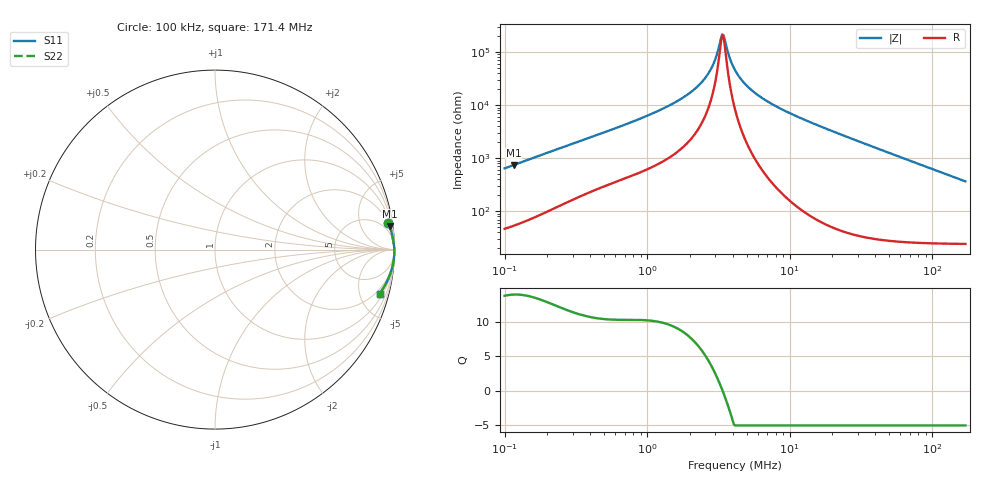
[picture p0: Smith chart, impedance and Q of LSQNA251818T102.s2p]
! LSQNA251818T102  S-PARAMETER MODEL  ( General Type )
! Model Generated by TAIYO YUDEN Corporation (http://www.ty-top.com)
! Version 2.0
! TAIYO YUDEN Control No. 100810NF25SB-FKC
! Copyright(c) 2007 TAIYO YUDEN CO.,LTD. All Rights Reserved.
! Product Description (link to TY-COMPAS)
! https://ds.yuden.co.jp/TYCOMPAS/or/detail?pn=LSQNA251818T102K&u=M
! Products Name : Inductors
! Characteristics :
!  Inductance : 1000 uH , SRF(min) : 2.4 MHz , DC Resistance(max) : 31.2 Ohm
!  Rated Current : Saturation :25 mA , Temp Rise : 75 mA (40 degC)
!  Case Size : 2.5 x 1.8 / 0.098 x 0.071 [mm/inch] , Thickness : 1.8 / 0.071 [mm/inch]
!  (Conditions: Temperature = 25 degC , DC Bias Current/Voltage = 0A / 0V)
! External Node Assignments :
!  1  o---GGG---o  2
! GND o---------o GND
! Frequency Range : 0.1MHz  -  171.398534MHz  [ 402 STEP ]
# MHz S RI R 50
! Freq[MHz].  S11 Real  S11 Imag  S21 Real  S21 Imag  S12 Real  S12 Imag  S22 Real  S22 Imag
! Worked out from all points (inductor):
!   401 points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, 100 kHz to 171.4 MHz, reference 50 ohm
!   read as one part in series: L = 1.02 mH near 103.8 kHz
!   highest Q = 13.9 at 116.1 kHz (marker M1), where L = 1.02 mH
!   self-resonance near 3.373 MHz
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0.1  0.9662 0.1479  0.0338 -0.1479  0.0338 -0.1479  0.9662 0.1479
0.116059  0.9734 0.1289  0.0266 -0.1289  0.0266 -0.1289  0.9734 0.1289
0.348094  0.9937 0.0455  0.00627 -0.0455  0.00627 -0.0455  0.9937 0.0455
1.211692  0.9986 0.0125  0.00142 -0.0125  0.00142 -0.0125  0.9986 0.0125
1.859293  0.9991 0.00668  0.000853 -0.00668  0.000853 -0.00668  0.9991 0.00668
2.157883  0.9993 0.00492  0.000721 -0.00492  0.000721 -0.00492  0.9993 0.00492
2.458233  0.9994 0.00346  0.000626 -0.00346  0.000626 -0.00346  0.9994 0.00346
2.698039  0.9994 0.00244  0.000569 -0.00244  0.000569 -0.00244  0.9994 0.00244
2.90662  0.9995 0.00164  0.000529 -0.00164  0.000529 -0.00164  0.9995 0.00164
3.073571  0.9995 0.00104  0.000503 -0.00104  0.000503 -0.00104  0.9995 0.00104
3.250112  0.9995 0.000449  0.000479 -0.000449  0.000479 -0.000449  0.9995 0.000449
3.373404  0.9995 5.2e-05  0.000464 -5.2e-05  0.000464 -5.2e-05  0.9995 5.2e-05
3.501373  0.9995 -0.000345  0.000451 0.000345  0.000451 0.000345  0.9995 -0.000345
3.842939  0.9996 -0.00134  0.000422 0.00134  0.000422 0.00134  0.9996 -0.00134
4.140031  0.9996 -0.00215  0.000403 0.00215  0.000403 0.00215  0.9996 -0.00215
4.895181  0.9996 -0.00403  0.000377 0.00403  0.000377 0.00403  0.9996 -0.00403
6.235538  0.9996 -0.00697  0.000374 0.00697  0.000374 0.00697  0.9996 -0.00697
8.717747  0.9995 -0.0118  0.00045 0.0118  0.00045 0.0118  0.9995 -0.0118
14.41119  0.9992 -0.0217  0.000836 0.0217  0.000836 0.0217  0.9992 -0.0217
50.16444  0.992 -0.0789  0.00803 0.0789  0.00803 0.0789  0.992 -0.0789
101.7716  0.9684 -0.1558  0.0316 0.1558  0.0316 0.1558  0.9684 -0.1558
171.3985  0.9167 -0.2451  0.0833 0.2451  0.0833 0.2451  0.9167 -0.2451
